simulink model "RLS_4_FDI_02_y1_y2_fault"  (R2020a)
settings: Solver=VariableStepAuto  StartTime=0.0  StopTime=30  RelTol=1e-3
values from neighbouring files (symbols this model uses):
  C = 6.3000e-04    (= 0.00063)    [maglev_init.m]
  g = 9.80    (= 9.8)    [maglev_init.m]
  K = 1.0e+03 * [-2.4567   -0.1235    0.0237]    [maglev_init.m]
  L1 = 0.6000    (= 0.6)    [maglev_init.m]
  m = 0.0300    (= 0.03)    [maglev_init.m]
  mpert = 0    [maglev_init.m]
  R = 45    [maglev_init.m]
  Ts = 0.005    [maglev_init.m]    (also in train_net.m)
  x1_0 = 0.1    [maglev_init.m]
  x1_d = 0.05    [maglev_init.m]
  x2_0 = 0    [maglev_init.m]
  x2_d = 0    [maglev_init.m]
  x3_0 = 0.2    [maglev_init.m]
undefined symbols (not defined in the file or in its folder): magnitude
libraries: ctrlSharedLib x2

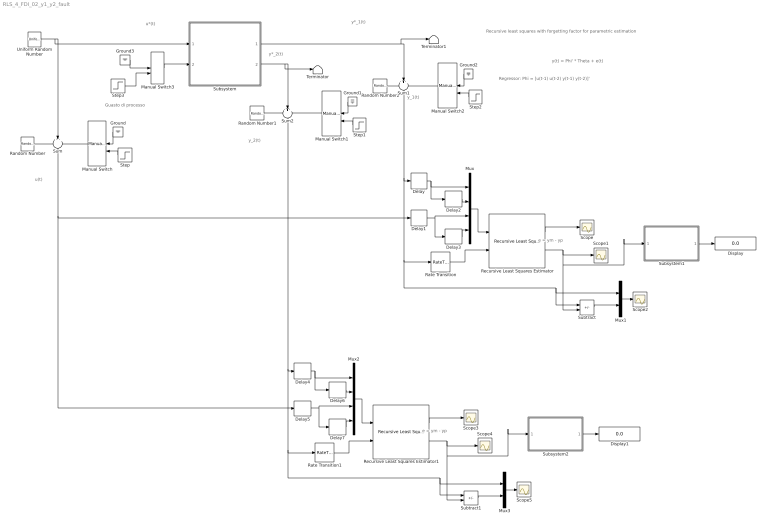
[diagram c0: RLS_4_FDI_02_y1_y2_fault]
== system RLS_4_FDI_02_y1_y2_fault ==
  note: Regressor: Phi = [u(t-1) u(t-2) y(t-1) y(t-2)]'
  note: y(t) = Phi' * Theta + e(t)
  note: Recursive least squares with forgetting factor for parametric estimation
  note: e = ym - yp
  note: y_2(t)
  note: y*_1(t)
  note: u(t)
  note: y*_2(t)
  note: y_1(t)
  note: u*(t)
  note: Guasto di processo
  note: e = ym - yp
  Delay{,1..7} (8 alike) : Delay  DelayLength=1  SampleTime=Ts
  Display : Display
  Display1 : Display
  Ground{,1..3} (4 alike) : Ground
  Manual Switch : ManualSwitch
  Manual Switch1 : ManualSwitch
  Manual Switch2 : ManualSwitch
  Manual Switch3 : ManualSwitch  CurrentSetting=0
  Mux : Mux
  Mux1 : Mux  Inputs=2
  Mux2 : Mux
  Mux3 : Mux  Inputs=2
  Random Number : RandomNumber  Variance=1e-9  Seed=1  SampleTime=Ts
  Random Number1 : RandomNumber  Variance=1e-6  Seed=3  SampleTime=Ts
  Random Number2 : RandomNumber  Variance=1e-9  Seed=2  SampleTime=Ts
  Rate Transition : RateTransition  OutPortSampleTime=Ts
  Rate Transition1 : RateTransition  OutPortSampleTime=Ts
  Recursive Least Squares Estimator : ctrlSharedLib/Recursive Least Squares Estimator  InitialEstimateSource=None  InitialParameterData=4  P0=1e4  InitialRegressors=0  InitialOutputs=0  History=Infinite  WindowLength=200  EstimationMethod=Forgetting Factor  AdaptationParameter=0.97  HasTimeVaryingAdaptationParameter=off  NormalizationBias=eps  OutputError=on  OutputP=off  AddEnablePort=off  InputProcessing=Sample-based  Ts=Ts
  Recursive Least Squares Estimator1 : ctrlSharedLib/Recursive Least Squares Estimator  InitialEstimateSource=None  InitialParameterData=4  P0=1e4  InitialRegressors=0  InitialOutputs=0  History=Infinite  WindowLength=200  EstimationMethod=Forgetting Factor  AdaptationParameter=0.97  HasTimeVaryingAdaptationParameter=off  NormalizationBias=eps  OutputError=on  OutputP=off  AddEnablePort=off  InputProcessing=Sample-based  Ts=Ts
  Scope{,1..5} (6 alike) : Scope
  Step : Step  Time=150  SampleTime=0
  Step1 : Step  Time=150  SampleTime=0
  Step2 : Step  Time=150  SampleTime=0
  Step3 : Step  Time=15  After=2*R  SampleTime=0
  Subsystem : Subsystem
  Subsystem1 : Subsystem
  Subsystem2 : Subsystem
  Subtract : Sum  Inputs=+-
  Subtract1 : Sum  Inputs=+-
  Sum : Sum  Inputs=+++
  Sum1 : Sum  Inputs=+++
  Sum2 : Sum  Inputs=+++
  Terminator : Terminator
  Terminator1 : Terminator
  Uniform Random Number : UniformRandomNumber  Minimum=x1_d*0.9  Maximum=x1_d*1.1  Seed=1  SampleTime=0.5
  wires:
  Subsystem/1(Out1) -> Terminator1/1, Sum1/2
  Subsystem/2(Out2) -> Terminator/1, Sum2/2
  Random Number/1 -> Sum/1
  Manual Switch/1 -> Sum/3
  Manual Switch2/1 -> Sum1/3
  Manual Switch1/1 -> Sum2/3
  Random Number1/1 -> Sum2/1
  Sum/1 -> Delay5/1, Delay1/1
  Ground/1 -> Manual Switch/1
  Step/1 -> Manual Switch/2
  Ground1/1 -> Manual Switch1/1
  Step1/1 -> Manual Switch1/2
  Random Number2/1 -> Sum1/1
  Ground2/1 -> Manual Switch2/1
  Step2/1 -> Manual Switch2/2
  Sum1/1 -> Mux1/1, Subtract/1, Rate Transition/1, Delay/1
  Mux/1 -> Recursive Least Squares Estimator/1
  Rate Transition/1 -> Recursive Least Squares Estimator/2
  Recursive Least Squares Estimator/1 -> Scope/1
  Recursive Least Squares Estimator/2 -> Subsystem1/1(e(t)), Subtract/2, Scope1/1
  Subtract/1 -> Mux1/2
  Mux1/1 -> Scope2/1
  Delay2/1 -> Mux/2
  Delay/1 -> Delay2/1, Mux/1
  Delay1/1 -> Delay3/1, Mux/3
  Delay3/1 -> Mux/4
  Subsystem1/1(RMS) -> Display/1
  Manual Switch3/1 -> Subsystem/2(fs)
  Ground3/1 -> Manual Switch3/1
  Uniform Random Number/1 -> Subsystem/1(u), Sum/2
  Step3/1 -> Manual Switch3/2
  Mux3/1 -> Scope5/1
  Delay7/1 -> Mux2/4
  Delay6/1 -> Mux2/2
  Subtract1/1 -> Mux3/2
  Mux2/1 -> Recursive Least Squares Estimator1/1
  Delay5/1 -> Delay7/1, Mux2/3
  Recursive Least Squares Estimator1/1 -> Scope3/1
  Recursive Least Squares Estimator1/2 -> Subsystem2/1(e(t)), Subtract1/2, Scope4/1
  Subsystem2/1(RMS) -> Display1/1
  Rate Transition1/1 -> Recursive Least Squares Estimator1/2
  Sum2/1 -> Mux3/1, Subtract1/1, Rate Transition1/1, Delay4/1
  Delay4/1 -> Delay6/1, Mux2/1

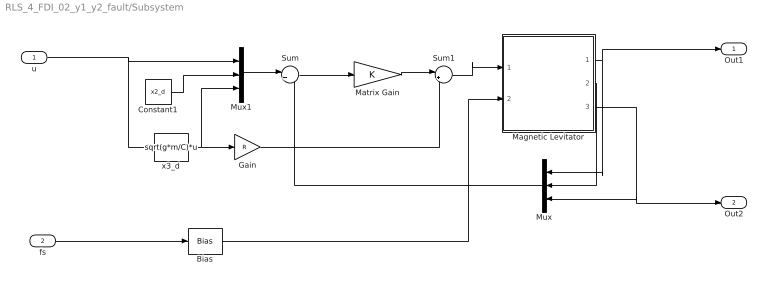
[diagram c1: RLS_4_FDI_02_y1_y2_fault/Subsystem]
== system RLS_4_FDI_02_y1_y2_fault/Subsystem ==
  u : Inport
  fs : Inport  Port=2
  Bias : Bias  Bias=R
  Constant1 : Constant  Value=x2_d
  Gain : Gain  Gain=R
  Magnetic Levitator : Subsystem  mask{m=m+mpert, R=R, L1=L1, C=C, g=g}
      mask prompts: m "ball's mass (m)"; R "Electromagnet's resistance (R)"; L1 "Electromagnet's inductance (L1)"; C "Magnetic force constant (C)"; g "Gravitational acceleration (g)"
  Matrix Gain : Gain  Gain=K  Multiplication=Matrix(K*u)  SaturateOnIntegerOverflow=on
  Mux : Mux  Inputs=3
  Mux1 : Mux  Inputs=3
  Sum : Sum  Inputs=|+-  InputSameDT=on  SaturateOnIntegerOverflow=on
  Sum1 : Sum  Inputs=|++  InputSameDT=on  SaturateOnIntegerOverflow=on
  x3_d : Fcn  Expr=sqrt(g*m/C)*u
  Out1 : Outport
  Out2 : Outport  Port=2
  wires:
  u/1 -> x3_d/1, Mux1/1
  Magnetic Levitator/2(x2) -> Mux/2
  x3_d/1 -> Mux1/3, Gain/1
  Mux1/1 -> Sum/1
  Gain/1 -> Sum1/2
  Mux/1 -> Sum/2
  Constant1/1 -> Mux1/2
  Sum/1 -> Matrix Gain/1
  Sum1/1 -> Magnetic Levitator/1(u)
  Magnetic Levitator/1(x1) -> Out1/1, Mux/1
  Magnetic Levitator/3(x3) -> Out2/1, Mux/3
  Matrix Gain/1 -> Sum1/1
  Bias/1 -> Magnetic Levitator/2(fs)
  fs/1 -> Bias/1

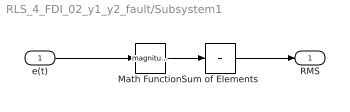
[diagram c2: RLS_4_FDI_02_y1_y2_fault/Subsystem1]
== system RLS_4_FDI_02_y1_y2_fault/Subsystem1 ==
  e(t) : Inport
  Math Function : Math  Operator=magnitude^2
  Sum of Elements : Sum  Inputs=+
  RMS : Outport
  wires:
  Math Function/1 -> Sum of Elements/1
  Sum of Elements/1 -> RMS/1
  e(t)/1 -> Math Function/1

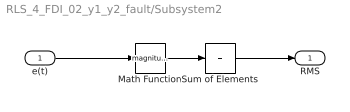
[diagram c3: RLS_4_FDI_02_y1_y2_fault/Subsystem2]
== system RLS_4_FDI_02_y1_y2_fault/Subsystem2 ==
  e(t) : Inport
  Math Function : Math  Operator=magnitude^2
  Sum of Elements : Sum  Inputs=+
  RMS : Outport
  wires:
  Math Function/1 -> Sum of Elements/1
  Sum of Elements/1 -> RMS/1
  e(t)/1 -> Math Function/1

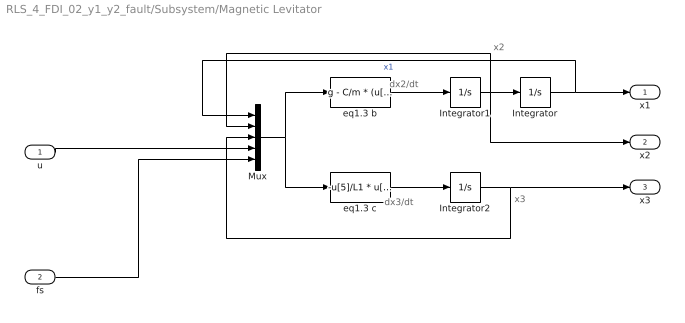
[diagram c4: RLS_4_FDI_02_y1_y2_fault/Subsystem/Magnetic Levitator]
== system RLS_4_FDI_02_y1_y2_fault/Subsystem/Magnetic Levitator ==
  note: x2
  note: x3
  note: dx2/dt
  note: dx3/dt
  u : Inport
  fs : Inport  Port=2
  Integrator : Integrator  InitialCondition=x1_0
  Integrator1 : Integrator  InitialCondition=x2_0
  Integrator2 : Integrator  InitialCondition=x3_0
  Mux : Mux  Inputs=5
  eq1.3 b : Fcn  Expr=g - C/m * (u[3] / u[1])^2
  eq1.3 c : Fcn  Expr=-u[5]/L1 * u[3] + (2*C)/L1 * ( u[2] * u[3] / u[1]^2 ) + 1/L1 * u[4]
  x1 : Outport
  x2 : Outport  Port=2
  x3 : Outport  Port=3
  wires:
  eq1.3 b/1 -> Integrator1/1
  Integrator1/1 -> Integrator/1, Mux/2, x2/1
  eq1.3 c/1 -> Integrator2/1
  Mux/1 -> eq1.3 b/1, eq1.3 c/1
  Integrator/1 -> Mux/1, x1/1  "x1"
  Integrator2/1 -> Mux/3, x3/1
  u/1 -> Mux/4
  fs/1 -> Mux/5
